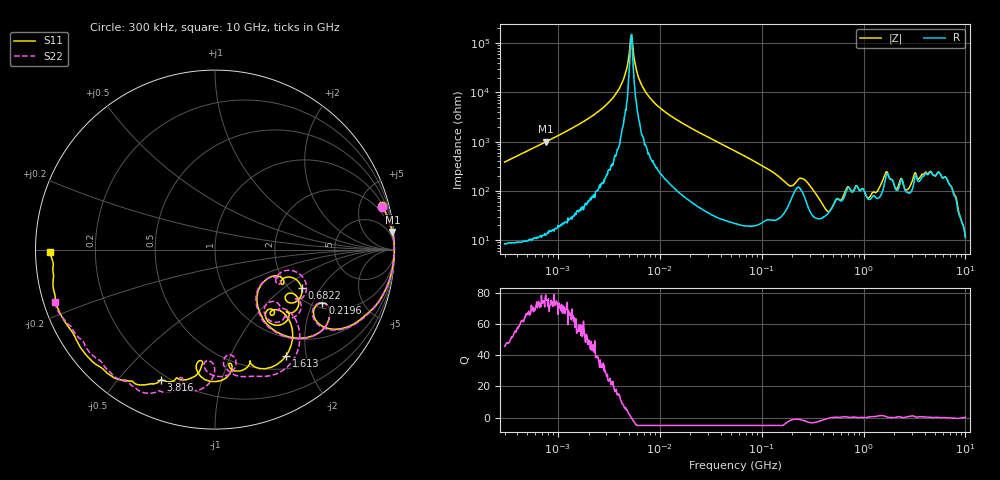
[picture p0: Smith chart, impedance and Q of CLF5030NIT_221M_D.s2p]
! S-Parameter Data Generated by TDK Corporation
! Copyright(C) 2019 TDK Corporation.
! All Rights Reserved.
! TDK P/N: CLF5030NIT-221M-D (Inductor)
! Property: L=220uH at 100kHz
! Size(LxWxT): 5.3x5x2.7mm
! Model Type: s2p (Touchstone File Format Version 1.0)
! Frequency: DC=Yes Start=0.3MHz Stop=10000MHz 802points Log-sweep
! Model Generated on May 10, 2019
! Port Assignments:
!  1 ---@@@--- 2
! Applicable Conditions:
!  Temperature = 25 degC
!  DC Bias Current = 0 A
!  Small Signal Operation
! Terms and conditions regarding TDK Simulation Models
! (1)This simulation model is being provided solely for informational purposes. Please refer to the specifications of the products in terms of detailed characteristics of such products.
! (2)In no event shall TDK Corporation of any of its subsidiaries be liable for any loss or damage arising, directly or indirectly,
!  From any information contained in this simulation model, including, but not limited to loss or damages arising from any inaccuracies, omissions or errors in connection with such information.
! (3)Any and all copyrights on this simulation model are owned by TDK Corporation.
!  Duplication or redistribution of this simulation model without prior written permission from TDK Corporation is prohibited.
! (4)This simulation model is subject to any modification or change without any prior notice.
! (5)Neither TDK Corporation nor any of its subsidiaries shall make any warranty, express or implied,
!  Including but not limited to the correctness, implied warranties of merchantability and fitness for a particular purpose with respect to this simulation models.
! (6)The use of this simulation model shall be deemed to have consented to the terms and conditions hereof.
# Hz S MA R 50
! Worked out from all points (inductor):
!   801 points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, 300 kHz to 10 GHz, reference 50 ohm
!   read as one part in series: L = 203 uH near 318.3 kHz
!   highest Q = 75.2 at 768.5 kHz (marker M1), where L = 207 uH
!   self-resonance near 5.231 MHz
!   S11 on the Smith chart (normalised r, x): 300 kHz: 1.19, +7.70; 219.6 MHz: 2.22, -2.38; 682.2 MHz: 2.29, -1.38; 1.613 GHz: 0.69, -1.65; 3.816 GHz: 0.17, -0.65; 10 GHz: 0.04, -0.01
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300000  0.9622 14.5  0.2501 -74.3  0.25 -74.3  0.9618 14.5
768539  0.9933 5.7  0.09941 -83.6  0.09941 -83.5  0.9932 5.7
1713600  0.9983 2.3  0.04102 -86.7  0.04101 -86.6  0.9982 2.3
3822232  0.9993 0.4  0.009769 -85.7  0.009765 -85.9  0.9993 0.4
4611084  0.9993 0.0  0.004027 -79.5  0.004013 -81.4  0.9994 0.0
5230511  0.9993 -0.2  0.0007086 -15.8  0.0007064 -12.7  0.9993 -0.2
6556275  0.9993 -0.6  0.006674 83.4  0.006592 82.6  0.9991 -0.6
9671944  0.9989 -1.5  0.01924 85.7  0.01925 85.6  0.9988 -1.5
5.477226e7  0.9832 -11.0  0.1518 77.1  0.1518 77.1  0.9833 -11.0
1.540638e8  0.8288 -32.1  0.4436 48.6  0.4436 48.6  0.8289 -32.5
2.195581e8  0.6684 -26.4  0.4146 19.6  0.4146 19.6  0.6644 -26.4
3.126428e8  0.693 -45.4  0.5602 29.0  0.5601 29.0  0.6923 -45.8
4.388767e8  0.363 -50.0  0.7177 -2.3  0.7176 -2.3  0.3594 -50.6
6.821612e8  0.5291 -24.1  0.4736 -35.0  0.4736 -35.0  0.5233 -18.3
1.10164e9  0.4621 -52.6  0.5426 -37.1  0.5426 -37.1  0.4338 -51.0
1.387199e9  0.4936 -43.4  0.507 -67.8  0.5071 -67.8  0.5098 -40.4
1.613252e9  0.7118 -56.2  0.2912 -88.3  0.2914 -88.3  0.7308 -51.1
1.767019e9  0.6731 -72.3  0.249 -65.0  0.249 -65.0  0.7603 -68.2
2.720446e9  0.6377 -96.2  0.31 -95.2  0.3102 -95.2  0.6212 -94.3
3.816223e9  0.785 -112.5  0.129 -114.7  0.1283 -114.7  0.8 -104.9
6.010849e9  0.9127 -133.6  0.0759 -121.6  0.07647 -121.4  0.8898 -135.6
1e10  0.9201 -179.0  0.05569 -93.3  0.0557 -93.6  0.9371 -161.9
